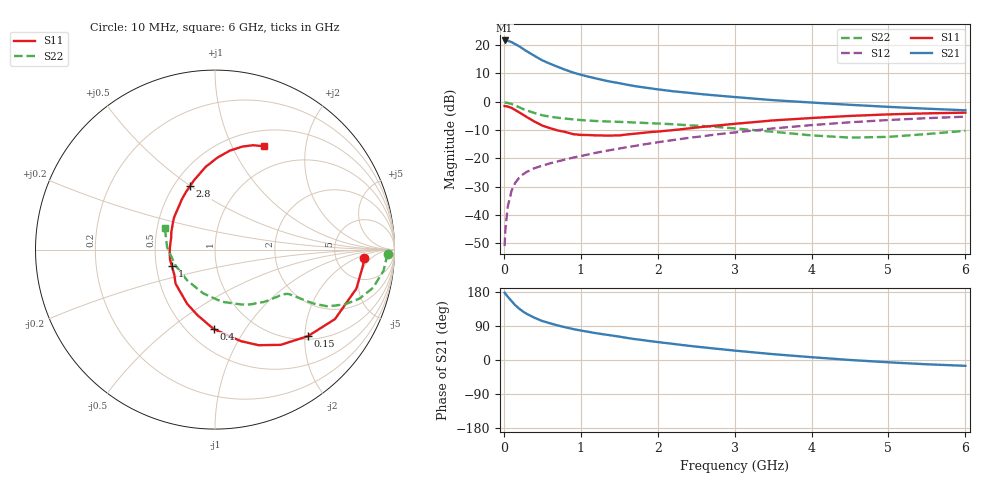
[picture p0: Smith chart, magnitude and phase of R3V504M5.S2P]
! SIEMENS Small Signal Semiconductors
! BFR181
! Si NPN RF Bipolar Junction Transistor in SOT23
! VCE = 0.5 V  IC = 4.5 mA
! Common Emitter S-Parameters:  May  1996
# GHz  S  MA  R  50
!  f  S11  S21  S12  S22
! GHz  MAG  ANG  MAG  ANG  MAG  ANG  MAG  ANG
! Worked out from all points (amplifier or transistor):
!   36 points, 10 MHz to 6 GHz, reference 50 ohm
!   highest |S21| = 21.6 dB at 10 MHz (marker M1)
!   |S21| within 3 dB of that: start of sweep to 251.2 MHz
!   unconditionally stable (mu >= 1): 686.5 MHz to end of sweep
!   at 250 MHz: K = 0.51, MSG = 22.1 dB, |S12| = -25.7 dB
!   at 1.4 GHz: K = 1.25, MAG = 9.0 dB, |S12| = -17.1 dB
!   at 6 GHz: K = 1.04, MAG = -0.1 dB, |S12| = -5.3 dB
!   S11 on the Smith chart (normalised r, x): 10 MHz: 10, -3; 150 MHz: 1.07, -2.07; 400 MHz: 0.66, -0.73; 1 GHz: 0.60, -0.12; 2.8 GHz: 0.60, +0.50; 6 GHz: 0.69, +1.34
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0.01  0.8325 -3.2  11.98 177.6  0.0028 86.9  0.962 -1.4
0.02  0.8295 -6.0  11.78 174.8  0.0054 85.3  0.9566 -3.0
0.05  0.8173 -15.4  11.81 167.3  0.0138 83.6  0.9463 -7.1
0.1  0.7724 -30.1  11.21 155.5  0.0266 75.1  0.9059 -13.6
0.15  0.7073 -43.0  10.3 144.3  0.0371 68.0  0.8504 -18.7
0.2  0.6447 -55.4  9.435 135.4  0.0453 63.1  0.7924 -22.4
0.25  0.5853 -65.5  8.5 127.8  0.0521 59.0  0.7365 -25.1
0.3  0.53 -74.2  7.695 121.5  0.0575 57.4  0.6966 -26.9
0.4  0.4426 -91.0  6.384 111.3  0.0667 54.5  0.6264 -28.7
0.5  0.3769 -105.3  5.339 102.9  0.0737 53.9  0.5734 -29.5
0.6  0.3397 -117.1  4.653 96.9  0.0811 53.9  0.5401 -29.9
0.7  0.3089 -127.6  4.1 91.2  0.0879 54.2  0.518 -30.3
0.8  0.2899 -139.4  3.63 86.3  0.0949 54.3  0.5003 -30.6
1  0.2577 -159.1  2.976 77.8  0.1092 55.6  0.472 -31.5
1.1  0.2562 -168.1  2.743 74.3  0.1167 56.0  0.4623 -32.4
1.6  0.2624 158.0  1.985 58.3  0.1568 56.6  0.4335 -37.7
2.2  0.3132 130.2  1.519 42.5  0.209 54.7  0.3976 -47.4
2.8  0.3808 111.3  1.268 29.0  0.2664 50.8  0.3531 -60.4
3.5  0.4643 96.4  1.058 15.4  0.3354 44.2  0.2931 -82.5
4.5  0.5575 81.5  0.876 0.1  0.4304 32.0  0.2312 -132.3
5.5  0.6189 70.0  0.748 -11.3  0.5088 18.9  0.2669 177.3
6  0.6371 64.6  0.701 -15.4  0.5409 11.9  0.3049 156.5
